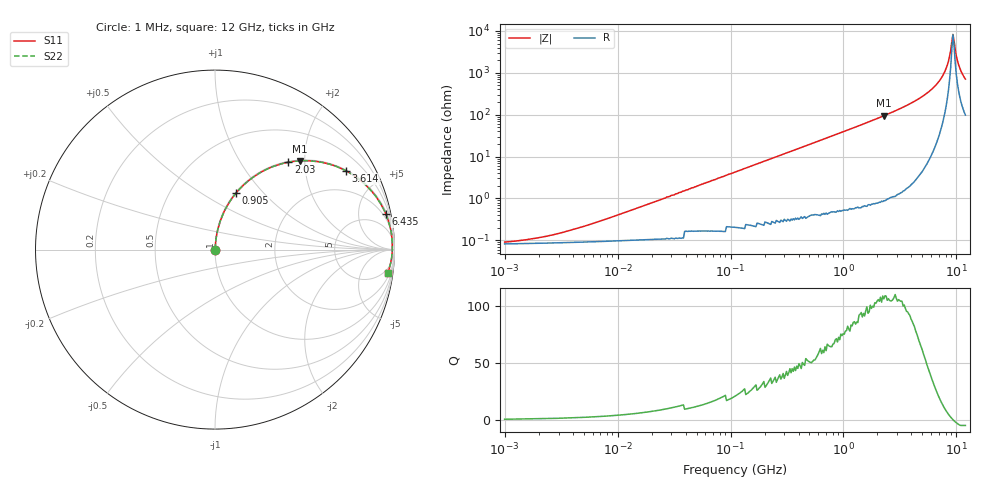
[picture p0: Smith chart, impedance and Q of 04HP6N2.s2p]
# MHz S MA R 50
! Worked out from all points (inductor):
!   408 points, 1 MHz to 12 GHz, reference 50 ohm
!   read as one part in series: L = 6.2 nH near 7.277 MHz
!   highest Q = 107 at 2.278 GHz (marker M1), where L = 6.59 nH
!   self-resonance near 9.31 GHz
!   S11 on the Smith chart (normalised r, x): 1 MHz: 1.00, +0.00; 905 MHz: 1.01, +0.71; 2.03 GHz: 1.02, +1.66; 3.614 GHz: 1.04, +3.31; 6.435 GHz: 1.34, +9.56; 12 GHz: 3, -14
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1  0.0007513 31.2  0.999 -0.0  0.999 -0.0  0.0007513 31.2
2.093  0.001078 49.0  0.999 -0.0  0.999 -0.0  0.001078 49.0
4.803  0.002039 66.4  0.999 -0.1  0.999 -0.1  0.002039 66.4
23.071  0.009054 82.0  0.999 -0.5  0.999 -0.5  0.009054 82.0
110.816  0.043 84.9  0.997 -2.5  0.997 -2.5  0.043 84.9
532.275  0.203 77.2  0.975 -11.7  0.975 -11.7  0.203 77.2
905.013  0.334 69.7  0.938 -19.5  0.938 -19.5  0.334 69.7
2029.758  0.636 50.0  0.766 -39.5  0.766 -39.5  0.636 50.0
2278.017  0.683 46.4  0.724 -43.1  0.724 -43.1  0.683 46.4
2556.642  0.729 42.6  0.677 -46.8  0.677 -46.8  0.729 42.6
3614.167  0.852 31.0  0.514 -58.5  0.514 -58.5  0.852 31.0
4992.568  0.934 20.0  0.343 -69.0  0.343 -69.0  0.934 20.0
6435.35  0.972 11.7  0.203 -76.3  0.203 -76.3  0.972 11.7
7222.457  0.982 8.0  0.14 -78.6  0.14 -78.6  0.982 8.0
7920.912  0.987 5.1  0.09 -78.9  0.09 -78.9  0.987 5.1
8488.733  0.988 2.9  0.053 -75.5  0.053 -75.5  0.988 2.9
9097.259  0.988 0.8  0.018 -48.8  0.018 -48.8  0.988 0.8
9309.645  0.988 0.1  0.012 -5.8  0.012 -5.8  0.988 0.1
9749.407  0.987 -1.4  0.027 59.6  0.027 59.6  0.987 -1.4
10209.94  0.985 -2.8  0.051 70.8  0.051 70.8  0.985 -2.8
10692.23  0.982 -4.2  0.075 73.9  0.075 73.9  0.982 -4.2
12000  0.972 -7.8  0.137 74.2  0.137 74.2  0.972 -7.8
